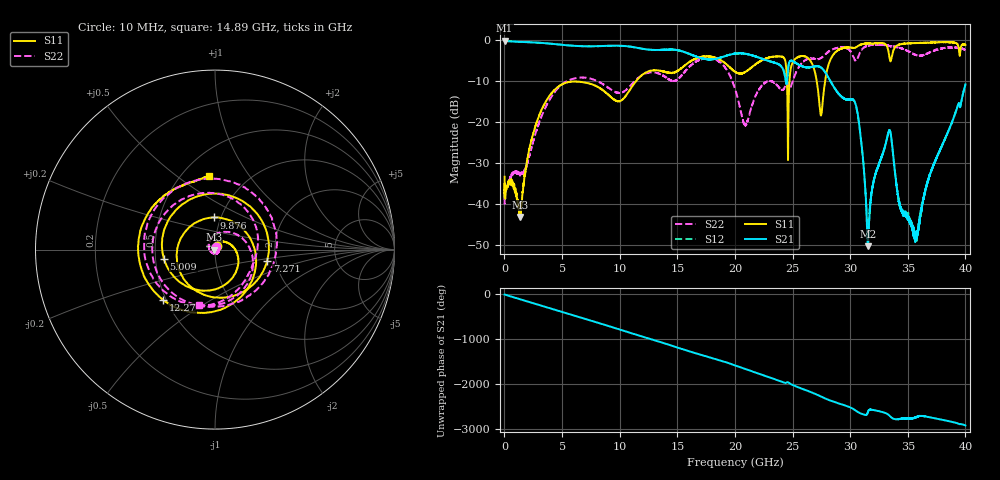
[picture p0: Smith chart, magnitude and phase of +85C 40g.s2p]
!Keysight Technologies,N5234A,MY52241180,A.10.60.03
!Date: Tuesday, February 27, 2024 09:09:37
!Correction: S11(Full 2 Port(1,2))
!S21(Full 2 Port(1,2))
!S12(Full 2 Port(1,2))
!S22(Full 2 Port(1,2))
!S2P File: Measurements: S11, S21, S12, S22:
# Hz S  dB  R 50
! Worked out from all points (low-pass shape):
!   6401 points, 10 MHz to 40 GHz, reference 50 ohm
!   highest |S21| = -0.07 dB at 10 MHz (marker M1); lowest = -50.4 dB at 31.55 GHz (marker M2)
!   |S21| within 3 dB of the highest: start of sweep to 15.78 GHz; 15.78165 GHz to 15.80325 GHz (21.61 MHz wide, 0.137 % of centre)
!   lowest |S11| = -43.2 dB at 1.385 GHz (marker M3), VSWR 1.01, Z = 49.3 - j0.0228 ohm
!   |S11| at or under -10 dB: start of sweep to 11.42 GHz; 24.51 GHz to 24.73 GHz (218.6 MHz wide, 0.888 % of centre); 27.1 GHz to 27.82 GHz (723.9 MHz wide, 2.64 % of centre)
!   |S22| runs from -40.0 to -1.0 dB; largest |S21 - S12| = 0.0086
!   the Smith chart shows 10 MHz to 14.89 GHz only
!   S11 on the Smith chart (normalised r, x): 10 MHz: 1.02, +0.04; 5.009 GHz: 0.55, -0.06; 7.271 GHz: 1.80, -0.24; 9.876 GHz: 0.93, +0.34; 12.27 GHz: 0.48, -0.32; 14.89 GHz: 0.67, +0.67
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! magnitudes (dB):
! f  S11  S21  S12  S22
! 10 MHz  -33.4  -0.1  -0.1  -35.9
! 1.385 GHz  -43.2  -0.4  -0.4  -32.6
! 2.809 GHz  -20.0  -0.6  -0.6  -21.8
! 5.009 GHz  -10.8  -1.1  -1.1  -10.8
! 6.677 GHz  -10.2  -1.5  -1.5  -9.1
! 7.271 GHz  -10.5  -1.5  -1.5  -9.3
! 9.876 GHz  -14.9  -1.3  -1.3  -12.9
! 12.27 GHz  -7.9  -2.2  -2.2  -8.1
! 13.34 GHz  -7.4  -2.4  -2.4  -8.1
! 14.89 GHz  -7.7  -2.4  -2.4  -9.9
! 17.94 GHz  -4.1  -4.7  -4.7  -4.4
! 20 GHz  -7.7  -3.3  -3.3  -11.9
! 20.93 GHz  -7.7  -3.3  -3.3  -20.9
! 26.67 GHz  -5.6  -6.5  -6.5  -4.5
! 27.47 GHz  -18.4  -6.7  -6.7  -4.3
! 28.43 GHz  -4.0  -10.7  -10.7  -2.3
! 30.43 GHz  -1.8  -15.3  -15.3  -4.9
! 31.55 GHz  -0.8  -50.4  -50.1  -1.3
! 33.34 GHz  -2.9  -22.3  -22.4  -1.3
! 34.33 GHz  -1.0  -41.0  -40.4  -1.9
! 35.68 GHz  -0.7  -47.6  -48.7  -3.6
! 40 GHz  -1.1  -10.8  -10.9  -2.4
